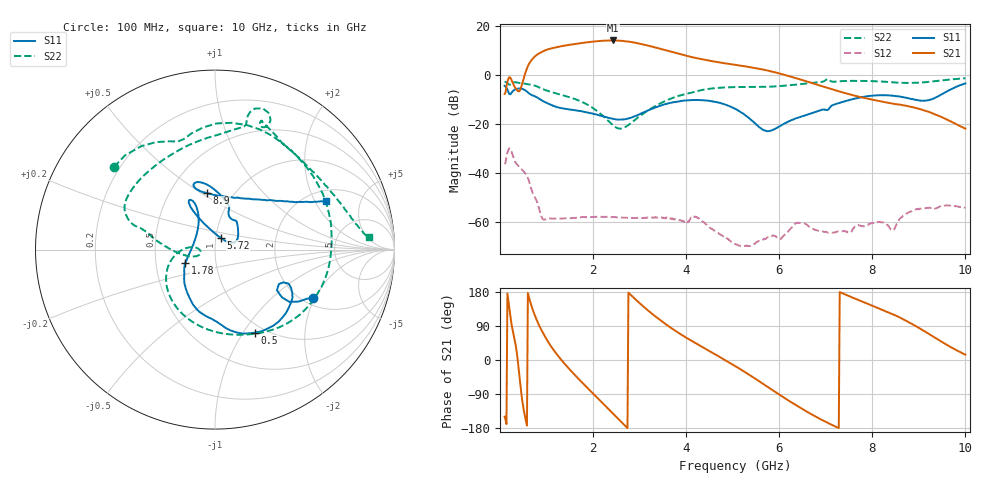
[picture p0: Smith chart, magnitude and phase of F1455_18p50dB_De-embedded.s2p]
! Integrated Device Technology
! Corporate Headquarters
! 6024 Silver Creek Valley Road
! San Jose, CA 95138  USA
! Phone:  1-408-284-8200
! Toll Free:  1-800-223-1366
! Webpage:  http://www.idt.com/
! Timing and RF Division
! 515 Groton Road, Suite 102
! Westford, MA 01886-6024
! Device:  F1455
! Description: 6-bit 0.5 dB Transmit Variable Gain Amplifier
! Frequency:  1400.0 -  2300.00 MHz
! Package:  6x6 mm Thin QFN Plastic Package: 28 pin
! State:  37
! Atten State:  18.5 dB
! Voltage:  +5.00 Volts
! Current:  217.623 mA
! Data:  The device was measured on a the F1455 evaluation board which has
!  individual transmission lines to the RF pins.  Data was collected
!  using a calibrated network analyzer.  The evaluation board was
!  de-embedded using a TRL calibration technique.
!  The reference plane is the edge of the package pin.
!  Pin  1 = CSb
!  Pin  2 = DATA
!  Pin  3 = CLK
!  Pin  4 = RSET
!  Pin  5 = GND
!  Pin  6 = RFIN  = Port 1
!  Pin  7 = GND
!  Pin  8 = NC
!  Pin  9 = NC
!  Pin 10 = NC
!  Pin 11 = NC
!  Pin 12 = NC
!  Pin 13 = NC
!  Pin 14 = /STBY
!  Pin 15 = GND
!  Pin 16 = RFOUT  = Port 2
!  Pin 17 = GND
!  Pin 18 = NC
!  Pin 19 = NC
!  Pin 20 = NC
!  Pin 21 = GND
!  Pin 22 = NC
!  Pin 23 = GND
!  Pin 24 = NC
!  Pin 25 = NC
!  Pin 26 = NC
!  Pin 27 = GND
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# GHz S dB R 50
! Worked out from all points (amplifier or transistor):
!   496 points, 100 MHz to 10 GHz, reference 50 ohm
!   highest |S21| = 14.1 dB at 2.42 GHz (marker M1)
!   |S21| within 3 dB of that: 1.158 GHz to 3.367 GHz (2.208 GHz wide, 97.6 % of centre)
!   unconditionally stable (mu >= 1): start of sweep to end of sweep
!   at 1.74 GHz: K = 77.99, MAG = 13.6 dB, |S12| = -58.0 dB
!   at 5.06 GHz: K = 567.36, MAG = 6.1 dB, |S12| = -69.1 dB
!   at 10 GHz: K = 434.82, MAG = -13.3 dB, |S12| = -54.1 dB
!   S11 on the Smith chart (normalised r, x): 100 MHz: 2.26, -1.92; 500 MHz: 0.90, -1.13; 1.78 GHz: 0.71, -0.11; 5.72 GHz: 1.06, +0.14; 8.9 GHz: 0.75, +0.53; 10 GHz: 2.47, +2.49
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0.1  -4.34 -26.2  -7.67 -149.6  -36.34 46.4  -2.77 140.7
0.26  -6.89 -24.8  -2.53 86.9  -31.93 -76.4  -3.31 95.7
0.38  -5.51 -41.8  -6.42 2.1  -36.76 -116.4  -3.08 57.8
0.5  -5.78 -64.1  -2.01 -123.8  -39.12 -155.0  -3.40 27.1
0.68  -8.10 -90.8  6.19 141.6  -46.84 139.9  -3.95 -14.5
0.82  -9.38 -109.0  8.62 96.9  -53.08 114.0  -4.81 -45.8
0.96  -10.95 -123.4  10.02 63.6  -58.95 125.3  -6.01 -71.2
1.34  -13.53 -144.4  11.87 -2.9  -58.57 94.3  -8.15 -121.5
1.76  -14.77 -155.7  13.11 -58.8  -57.95 61.9  -10.91 -158.4
1.78  -14.88 -156.2  13.16 -61.3  -57.92 59.8  -11.09 -159.9
2.1  -16.24 -166.0  13.86 -100.7  -57.80 42.3  -14.84 -179.9
2.42  -17.80 174.9  14.15 -140.4  -57.89 28.0  -20.33 175.8
2.8  -17.48 139.7  13.57 173.0  -58.26 15.0  -19.77 -160.5
3.1  -15.09 121.3  12.42 139.2  -58.23 7.9  -15.48 -169.4
3.4  -12.77 114.5  10.97 109.3  -58.05 -2.6  -12.00 179.0
4.08  -10.22 116.1  7.53 53.2  -58.96 -14.2  -7.32 163.8
5.06  -13.79 117.4  4.18 -16.4  -69.06 -44.0  -4.88 148.5
5.72  -22.79 63.2  2.00 -68.3  -66.69 -11.4  -4.78 121.3
6.7  -15.55 39.7  -3.21 -143.7  -62.40 -131.8  -3.20 78.6
8.36  -8.28 107.7  -11.38 124.5  -61.92 111.4  -2.82 62.5
8.9  -9.95 98.3  -13.24 91.7  -55.01 122.2  -3.16 41.0
10  -3.39 23.8  -21.84 14.1  -54.12 44.8  -1.29 4.6
